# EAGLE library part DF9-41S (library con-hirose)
SMD CONNECTOR Source: con-hirose.lbr from Bob Starr <rtzaudio@mindspring.com>
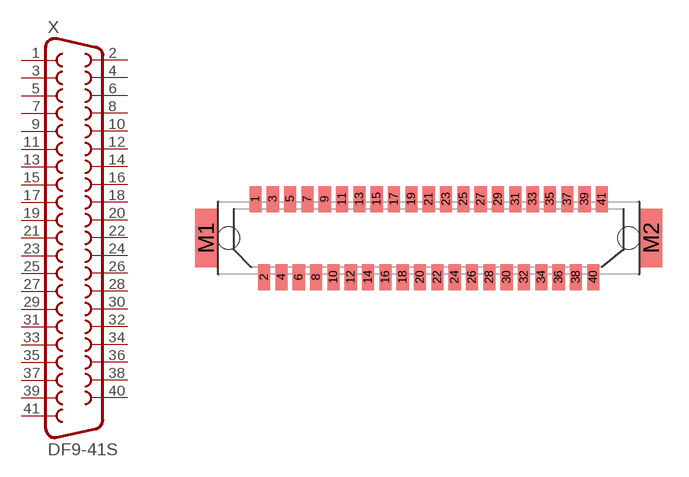
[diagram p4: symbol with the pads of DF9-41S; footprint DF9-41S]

Designator prefix X

## DF9-41S (MPN: DF9-41S-1V(32); OC_FARNELL: 1798384; OC_NEWARK: 74R3385)  [DF9-41S]
1  1  pas
2  2  pas
3  3  pas
4  4  pas
5  5  pas
6  6  pas
7  7  pas
8  8  pas
9  9  pas
10  10  pas
11  11  pas
12  12  pas
13  13  pas
14  14  pas
15  15  pas
16  16  pas
17  17  pas
18  18  pas
19  19  pas
20  20  pas
21  21  pas
22  22  pas
23  23  pas
24  24  pas
25  25  pas
26  26  pas
27  27  pas
28  28  pas
29  29  pas
30  30  pas
31  31  pas
32  32  pas
33  33  pas
34  34  pas
35  35  pas
36  36  pas
37  37  pas
38  38  pas
39  39  pas
40  40  pas
41  41  pas

## Footprint DF9-41S (pad centres in mm)
CONNECTOR
smd 0.7 x 1.5: 1 -10,2.25; 2 -9.5,-2.25; 3 -9,2.25; 4 -8.5,-2.25; 5 -8,2.25; 6 -7.5,-2.25; 7 -7,2.25; 8 -6.5,-2.25; 9 -6,2.25; 10 -5.5,-2.25; 11 -5,2.25; 12 -4.5,-2.25; 13 -4,2.25; 14 -3.5,-2.25; 15 -3,2.25; 16 -2.5,-2.25; 17 -2,2.25; 18 -1.5,-2.25; 19 -1,2.25; 20 -0.5,-2.25; 21 0,2.25; 22 0.5,-2.25; 23 1,2.25; 24 1.5,-2.25; 25 2,2.25; 26 2.5,-2.25; 27 3,2.25; 28 3.5,-2.25; 29 4,2.25; 30 4.5,-2.25; 31 5,2.25; 32 5.5,-2.25; 33 6,2.25; 34 6.5,-2.25; 35 7,2.25; 36 7.5,-2.25; 37 8,2.25; 38 8.5,-2.25; 39 9,2.25; 40 9.5,-2.25; 41 10,2.25
smd 1.3 x 3.4: M1 -12.85,0; M2 12.85,0
hole 1.27 at 11.55,0
hole 1.27 at -11.55,0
